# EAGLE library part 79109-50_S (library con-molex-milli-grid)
RECEPTACAL
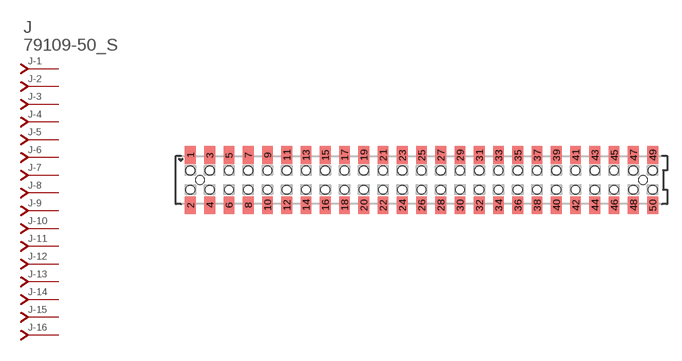
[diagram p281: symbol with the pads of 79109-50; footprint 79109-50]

Designator prefix J; gates -1=J-NV -2=J-N -3=J-N -4=J-N -5=J-N -6=J-N -7=J-N -8=J-N -9=J-N -10=J-N -11=J-N -12=J-N -13=J-N -14=J-N -15=J-N -16=J-N -17=J-N -18=J-N -19=J-N -20=J-N -21=J-N -22=J-N -23=J-N -24=J-N -25=J-N -26=J-N -27=J-N -28=J-N -29=J-N -30=J-N -31=J-N -32=J-N -33=J-N -34=J-N -35=J-N -36=J-N -37=J-N -38=J-N -39=J-N -40=J-N -41=J-N -42=J-N -43=J-N -44=J-N -45=J-N -46=J-N -47=J-N -48=J-N -49=J-N -50=J-N

## 79109-50_S  [79109-50]
1  -1:J  pas
2  -2:J  pas
3  -3:J  pas
4  -4:J  pas
5  -5:J  pas
6  -6:J  pas
7  -7:J  pas
8  -8:J  pas
9  -9:J  pas
10  -10:J  pas
11  -11:J  pas
12  -12:J  pas
13  -13:J  pas
14  -14:J  pas
15  -15:J  pas
16  -16:J  pas
17  -17:J  pas
18  -18:J  pas
19  -19:J  pas
20  -20:J  pas
21  -21:J  pas
22  -22:J  pas
23  -23:J  pas
24  -24:J  pas
25  -25:J  pas
26  -26:J  pas
27  -27:J  pas
28  -28:J  pas
29  -29:J  pas
30  -30:J  pas
31  -31:J  pas
32  -32:J  pas
33  -33:J  pas
34  -34:J  pas
35  -35:J  pas
36  -36:J  pas
37  -37:J  pas
38  -38:J  pas
39  -39:J  pas
40  -40:J  pas
41  -41:J  pas
42  -42:J  pas
43  -43:J  pas
44  -44:J  pas
45  -45:J  pas
46  -46:J  pas
47  -47:J  pas
48  -48:J  pas
49  -49:J  pas
50  -50:J  pas

## Footprint 79109-50 (pad centres in mm)
RECEPTACAL SMD Dual Row, Vertical, Pass-Thru
smd 1.12 x 1.83: 1 -24,2.6; 2 -24,-2.6; 3 -22,2.6; 4 -22,-2.6; 5 -20,2.6; 6 -20,-2.6; 7 -18,2.6; 8 -18,-2.6; 9 -16,2.6; 10 -16,-2.6; 11 -14,2.6; 12 -14,-2.6; 13 -12,2.6; 14 -12,-2.6; 15 -10,2.6; 16 -10,-2.6; 17 -8,2.6; 18 -8,-2.6; 19 -6,2.6; 20 -6,-2.6; 21 -4,2.6; 22 -4,-2.6; 23 -2,2.6; 24 -2,-2.6; 25 0,2.6; 26 0,-2.6; 27 2,2.6; 28 2,-2.6; 29 4,2.6; 30 4,-2.6; 31 6,2.6; 32 6,-2.6; 33 8,2.6; 34 8,-2.6; 35 10,2.6; 36 10,-2.6; 37 12,2.6; 38 12,-2.6; 39 14,2.6; 40 14,-2.6; 41 16,2.6; 42 16,-2.6; 43 18,2.6; 44 18,-2.6; 45 20,2.6; 46 20,-2.6; 47 22,2.6; 48 22,-2.6; 49 24,2.6; 50 24,-2.6
hole 0.914 at -23,0
hole 0.914 at -24,1
hole 0.914 at -24,-1
hole 0.914 at -22,-1
hole 0.914 at -22,1
hole 0.914 at -20,-1
hole 0.914 at -20,1
hole 0.914 at -18,1
hole 0.914 at -18,-1
hole 0.914 at -16,1
hole 0.914 at -16,-1
hole 0.914 at -14,1
hole 0.914 at -14,-1
hole 0.914 at -12,1
hole 0.914 at -12,-1
hole 0.914 at -10,-1
hole 0.914 at -10,1
hole 0.914 at -8,1
hole 0.914 at -8,-1
hole 0.914 at -6,1
hole 0.914 at -6,-1
hole 0.914 at -4,1
hole 0.914 at -4,-1
hole 0.914 at -2,-1
hole 0.914 at -2,1
hole 0.914 at 0,1
hole 0.914 at 2,1
hole 0.914 at 4,1
hole 0.914 at 0,-1
hole 0.914 at 2,-1
hole 0.914 at 4,-1
hole 0.914 at 6,-1
hole 0.914 at 8,-1
hole 0.914 at 10,-1
hole 0.914 at 12,-1
hole 0.914 at 14,-1
hole 0.914 at 6,1
hole 0.914 at 8,1
hole 0.914 at 10,1
hole 0.914 at 12,1
hole 0.914 at 14,1
hole 0.914 at 16,-1
hole 0.914 at 18,-1
hole 0.914 at 16,1
hole 0.914 at 18,1
hole 0.914 at 20,1
hole 0.914 at 22,1
hole 0.914 at 24,1
hole 0.914 at 20,-1
hole 0.914 at 22,-1
hole 0.914 at 24,-1
hole 0.914 at 23,0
